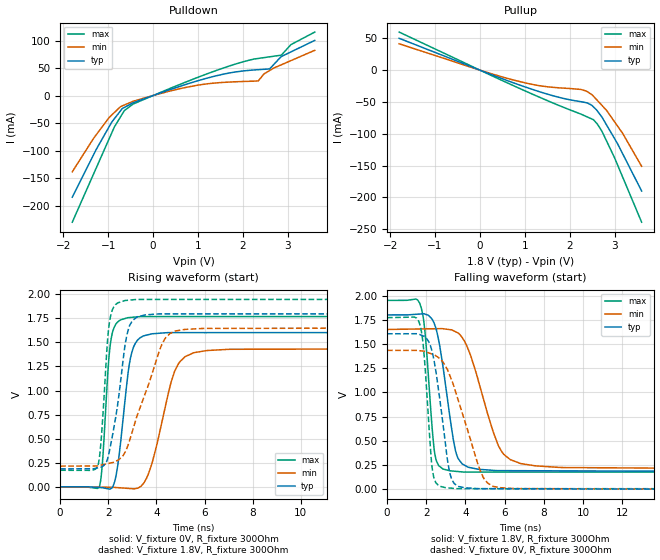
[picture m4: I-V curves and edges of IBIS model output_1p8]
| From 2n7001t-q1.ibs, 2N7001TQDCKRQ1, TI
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|   output_1p8 Model
[Model]   output_1p8
Model_type   Output
Polarity   Non-Inverting
Vmeas = 0.9
Vref = 0
Cref = 2pF
Rref = 100000
|   typ   min   max
C_comp   0.886pF   0.779pF   1.27pF
|  Where Nom  PVT is Nominal Process,   1.8V,  27C
|   Fast PVT is Strong Process,   1.95V, -40C
|   Slow PVT is Weak Process,   1.65V, 130C
[Voltage Range]   1.8   1.65   1.95
|Junction Temperature
[Temperature Range]   27   130   -40
[Pullup Reference]   1.8   1.65   1.95
[Pulldown Reference]   0   -0   -0
[Power Clamp Reference]   1.8   1.65   1.95
[GND Clamp Reference]   0   0   0
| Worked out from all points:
|   slope of the pulldown table from 0 to 0.27 V, typ, clamps not added: 34.8 ohm
|   slope of the pullup table from 0 to 0.27 V, typ, clamps not added: 36.5 ohm
|   falling waveform, V_fixture 1.8V, R_fixture 300Ohm: 20-80 % time 694ps typ, 1.29ns min, 398ps max; typ from 1.8 V to 0.186 V
|   rising waveform, V_fixture 0V, R_fixture 300Ohm: 20-80 % time 437ps typ, 824ps min, 270ps max; typ from 0 V to 1.6 V
|   rising waveform, V_fixture 1.8V, R_fixture 300Ohm: 20-80 % time 544ps typ, 1.15ns min, 279ps max; typ from 0.186 V to 1.8 V
|   falling waveform, V_fixture 0V, R_fixture 300Ohm: 20-80 % time 633ps typ, 1.33ns min, 359ps max; typ from 1.6 V to 0 V
[Pulldown]
|   Voltage   I(typ)   I(min)   I(max)
-1.8V     -184.8mA   -138.7mA   -230.3mA
-1.33V    -108.4mA   -78.37mA   -143.5mA
-918.3mV  -47.94mA   -35.15mA   -67.43mA
-641.6mV  -21.72mA   -17.23mA   -27.53mA
-449.9mV  -13.2mA    -10.59mA   -15.66mA
977mV     26.4mA     18.62mA    32.5mA
1.633V    40.01mA    24.19mA    51.9mA
2.342V    47.03mA    26.61mA    67.47mA
2.594V    48.34mA    45.46mA    70.41mA
2.856V    70.9mA     55.94mA    73.46mA
3.071V    79.39mA    63.54mA    92.68mA
3.6V      100.3mA    82.22mA    115.4mA
[Pullup]
|   Voltage   I(typ)   I(min)   I(max)
-1.8V     50.14mA    41.51mA    59.93mA
778.3mV   -20.75mA   -16.09mA   -25.42mA
1.324V    -33.87mA   -24.45mA   -42.52mA
2.25V     -49.58mA   -30.33mA   -69.16mA
2.393V    -51.63mA   -33.95mA   -73.71mA
2.527V    -57.77mA   -41.03mA   -77.98mA
2.615V    -64.34mA   -47.71mA   -84.84mA
2.717V    -73.97mA   -55.48mA   -96.35mA
2.814V    -85.64mA   -62.84mA   -110.7mA
2.994V    -107.3mA   -80.93mA   -137.3mA
3.177V    -131.5mA   -99.4mA    -168.1mA
3.6V      -190.1mA   -151.2mA   -239.2mA
[Ramp]
R_load = 300
|   typ   min   max
dV/dt_r   0.963238/4.35788e-10   0.860231/8.17571e-10   1.06317/2.69098e-10
dV/dt_f   0.96847/6.93404e-10   0.861348/1.28076e-09   1.06704/3.97377e-10
[Falling Waveform]
V_fixture = 1.8V
V_fixture_min = 1.65V
V_fixture_max = 1.95V
R_fixture = 300Ohm
C_fixture = 0F
|   Time   V(typ)   V(min)   V(max)
0s        1.8V       1.65V      1.95V
1.67ns    1.809V     1.655V     1.918V
1.925ns   1.809V     1.656V     1.642V
2.44ns    1.693V     1.657V     360mV
3.212ns   735.8mV    1.648V     189.7mV
3.494ns   394.5mV    1.626V     184.4mV
3.828ns   261.4mV    1.567V     178.2mV
5.794ns   191.6mV    404.4mV    177mV
7.549ns   190.3mV    241.2mV    177mV
50ns      185.9mV    214.4mV    171.6mV
[Rising Waveform]
V_fixture = 0V
V_fixture_min = 0V
V_fixture_max = 0V
R_fixture = 300Ohm
C_fixture = 0F
|   Time   V(typ)   V(min)   V(max)
0s        -18.2nV    -108.7nV   -63.42nV
1.619ns   -7.246mV   -3.991mV   -5.117mV
2.122ns   -16.32mV   -5.23mV    1.542V
2.392ns   220mV      -8.819mV   1.712V
2.802ns   1.139V     -16.24mV   1.756V
3.069ns   1.462V     -20.95mV   1.762V
3.677ns   1.581V     140.2mV    1.768V
4.922ns   1.601V     1.281V     1.768V
6.097ns   1.601V     1.415V     1.768V
50ns      1.605V     1.434V     1.772V
[Rising Waveform]
V_fixture = 1.8V
V_fixture_min = 1.65V
V_fixture_max = 1.95V
R_fixture = 300Ohm
C_fixture = 0F
|   Time   V(typ)   V(min)   V(max)
0s        185.9mV    214.4mV    171.6mV
1.559ns   196.2mV    217.2mV    213.4mV
1.699ns   203.7mV    225mV      471.7mV
1.962ns   283.7mV    239.7mV    1.497V
2.062ns   388.6mV    245.3mV    1.73V
2.694ns   1.467V     357.9mV    1.935V
3.004ns   1.727V     578.9mV    1.942V
4.215ns   1.796V     1.472V     1.946V
5.189ns   1.796V     1.635V     1.946V
50ns      1.8V       1.65V      1.95V
[Falling Waveform]
|Gnd
V_fixture = 0V
V_fixture_min = 0V
V_fixture_max = 0V
R_fixture = 300Ohm
C_fixture = 0F
|   Time   V(typ)   V(min)   V(max)
0s        1.605V     1.434V     1.772V
1.636ns   1.6V       1.431V     1.725V
1.871ns   1.581V     1.426V     1.433V
2.329ns   1.395V     1.393V     179mV
2.968ns   483.7mV    1.275V     15.83mV
3.187ns   178.8mV    1.181V     11.91mV
3.421ns   58.89mV    1.054V     7.73mV
4.896ns   5.002mV    125.7mV    4.977mV
5.757ns   4.551mV    15.56mV    4.955mV
50ns      5.57nV     102.5nV    46.29nV
